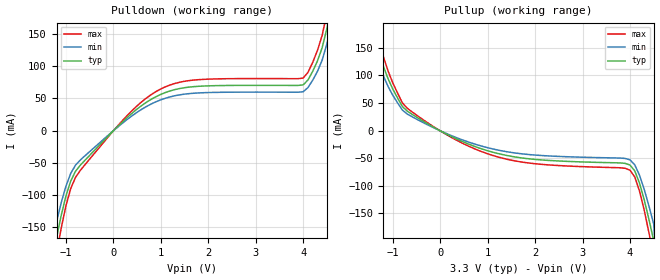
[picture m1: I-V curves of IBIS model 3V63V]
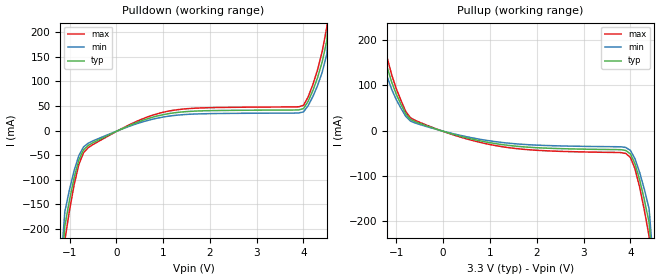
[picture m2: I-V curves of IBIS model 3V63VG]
[IBIS Ver]   2.1
[File name]   2703_3.ibs
[File Rev]   2.0
[Date]   8/2/01
[Source]   ICS MicroClock Applications Engineering 2
[Disclaimer] This information is for modeling purposes only, and is
(C) Copyright Integrated Circuit Systems, Inc. 1997-2001
   All rights reserved
ICS hereby grants the user of this IBIS model a non-exclusive,
nontransferable license to use this IBIS model under the following terms.
Before using this IBIS model, the user should read this license.
If the user does not accept these terms,  the IBIS model should be
returned to ICS within 30 days.
   The user is granted this license only to use the IBIS model and
is not granted rights to sell, load, rent, lease or license the IBIS
model in whole or in part, or in modified form to anyone other than
user. User may modify the IBIS model to suit its specific
applications but rights to derivative works and such modifications
shall belong to ICS.
   This IBIS model is provided on an "AS IS" basis and ICS makes
absolutely no warranty with respect to the information contained
herein. ICS DISCLAIMS AND CUSTOMER WAIVES ALL WARRANTIES, EXPRESS
OR IMPLIED, INCLUDING WARRANTIES OF MERCHANTABILITY OR FITNESS FOR
A PARTICULAR PURPOSE. The entire risk as to quality and performance
is with the Customer. ACCORDINGLY, IN NO EVENT SHALL THE COMPANY BE
LIABLE FOR ANY DAMAGES, WHETHER IN CONTRACT OR TORT,INCLUDING ANY
LOST PROFITS OR OTHER INCIDENTAL, CONSEQUENTIAL, EXEMPLARY, OR
PUNITIVE DAMAGES ARISING OUT OF THE USE OR APPLICATION OF THE IBIS
model provided in this package. Further, ICS reserves the right to
make changes without notice to any product herein to improve
reliability, function, or design. ICS does not convey any license
under patent rights or any other intellectual property rights,
including those of third parties.
   ICS is not obligated to provide maintenance or support
for the licensed IBIS model.
[Component]   Mk2703
[Manufacturer] Integrated Circuit Systems Inc.
[Package]
|   typ   min   max
R_pkg   40m   35m   45m
L_pkg   1.65nH   1.35nH   1.95nH
C_pkg   0.24pF   0.14pF   0.34pF
[pin]   signal_name   model_name   R_pin   L_pin   C_pin
   4   27M   3V63V
   5   CLK   3V63VG
| Models and submodels in the file (2): 3V63V (Output), 3V63VG (Output)
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|   MK2703  3.3V Clock Drive Model
| This model is suitable for 27M output pin on the
| MK2703
[Model]   3V63V
Model_type   Output
Polarity   Non-Inverting
|   typ   min   max
C_comp   5pF   4pF   6pF
|   typ   min   max
[Voltage range]  3.3V   3.15V   3.45V
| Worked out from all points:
|   slope of the pulldown table from 0 to 0.495 V, typ, clamps not added: 14.9 ohm
|   slope of the pullup table from 0 to 0.495 V, typ, clamps not added: 24.2 ohm
[pulldown]
|Voltage I (typ)   I (min)   I (max)
-3.3V     -3A        -3A        -3A
-1.3V     -199.9mA   -169.9mA   -229.9mA
-1.2V     -166.1mA   -141.2mA   -191mA
-1.1V     -131mA     -111.3mA   -150.6mA
-800mV    -63.14mA   -53.66mA   -72.61mA
400mV     27.29mA    23.2mA     31.39mA
1.1V      58.96mA    50.11mA    67.8mA
4V        70.65mA    60.05mA    81.25mA
4.3V      107.5mA    91.34mA    123.6mA
4.5V      157.8mA    134.1mA    181.5mA
4.6V      195.8mA    166.4mA    225.2mA
6.6V      3A         3A         3A
[pullup]
|Voltage I (typ)   I (min)   I (max)
-3.3V     3A         3A         3A
-1.4V     190.5mA    161.9mA    219.1mA
-1.3V     149.2mA    126.8mA    171.6mA
-1.2V     116.4mA    98.91mA    133.8mA
-800mV    43.62mA    37.08mA    50.17mA
400mV     -17.51mA   -14.88mA   -20.14mA
1.6V      -48.26mA   -41.02mA   -55.49mA
4V        -62.64mA   -53.25mA   -72.04mA
4.2V      -95.46mA   -81.14mA   -109.8mA
4.4V      -161.7mA   -137.4mA   -185.9mA
4.5V      -199.9mA   -169.9mA   -229.9mA
6.6V      -3A        -3A        -3A
[Ramp]
|   typ   min   max
dV/dt_r   1.31/0.41n   1.24/0.45n   1.37/0.37n
dV/dt_f   1.54/0.34n   1.46/0.38n   1.62/0.31n
|   MK2703  3.3V Clock Drive Model
| This model is suitable for  CLK output pin   on the
| MK2703
[Model]   3V63VG
Model_type   Output
Polarity   Non-Inverting
|   typ   min   max
C_comp   5pF   4pF   6pF
|   typ   min   max
[Voltage range]  3.3V   3.15V   3.45V
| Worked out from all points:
|   slope of the pulldown table from 0 to 0.495 V, typ, clamps not added: 24.7 ohm
|   slope of the pullup table from 0 to 0.495 V, typ, clamps not added: 34.9 ohm
[pulldown]
|Voltage I (typ)   I (min)   I (max)
-3.3V     -3A        -3A        -3A
-1.1V     -194mA     -164.9mA   -223.1mA
-900mV    -95.08mA   -80.82mA   -109.3mA
-800mV    -59.68mA   -50.73mA   -68.63mA
-700mV    -39.05mA   -33.19mA   -44.9mA
-500mV    -24.78mA   -21.06mA   -28.5mA
400mV     14.86mA    12.63mA    17.09mA
1.1V      33.99mA    28.89mA    39.09mA
4V        44.46mA    37.79mA    51.13mA
4.3V      107mA      90.95mA    123mA
4.5V      183.1mA    155.6mA    210.5mA
6.6V      3A         3A         3A
[pullup]
|Voltage I (typ)   I (min)   I (max)
-3.3V     3A         3A         3A
-1.3V     185.7mA    157.8mA    213.6mA
-1.2V     140.7mA    119.6mA    161.8mA
-1V       79.5mA     67.58mA    91.43mA
-800mV    36.6mA     31.11mA    42.09mA
-600mV    19.53mA    16.6mA     22.46mA
1.3V      -31.51mA   -26.78mA   -36.24mA
3.9V      -43.88mA   -37.3mA    -50.46mA
4V        -51.33mA   -43.63mA   -59.03mA
4.1V      -73.5mA    -62.47mA   -84.52mA
4.4V      -202.5mA   -172.1mA   -232.9mA
6.6V      -3A        -3A        -3A
[Ramp]
|   typ   min   max
dV/dt_r   1.06/0.92n   1.00/1.01n   1.11/0.83n
dV/dt_f   1.19/0.96n   1.13/1.06n   1.25/0.86n
